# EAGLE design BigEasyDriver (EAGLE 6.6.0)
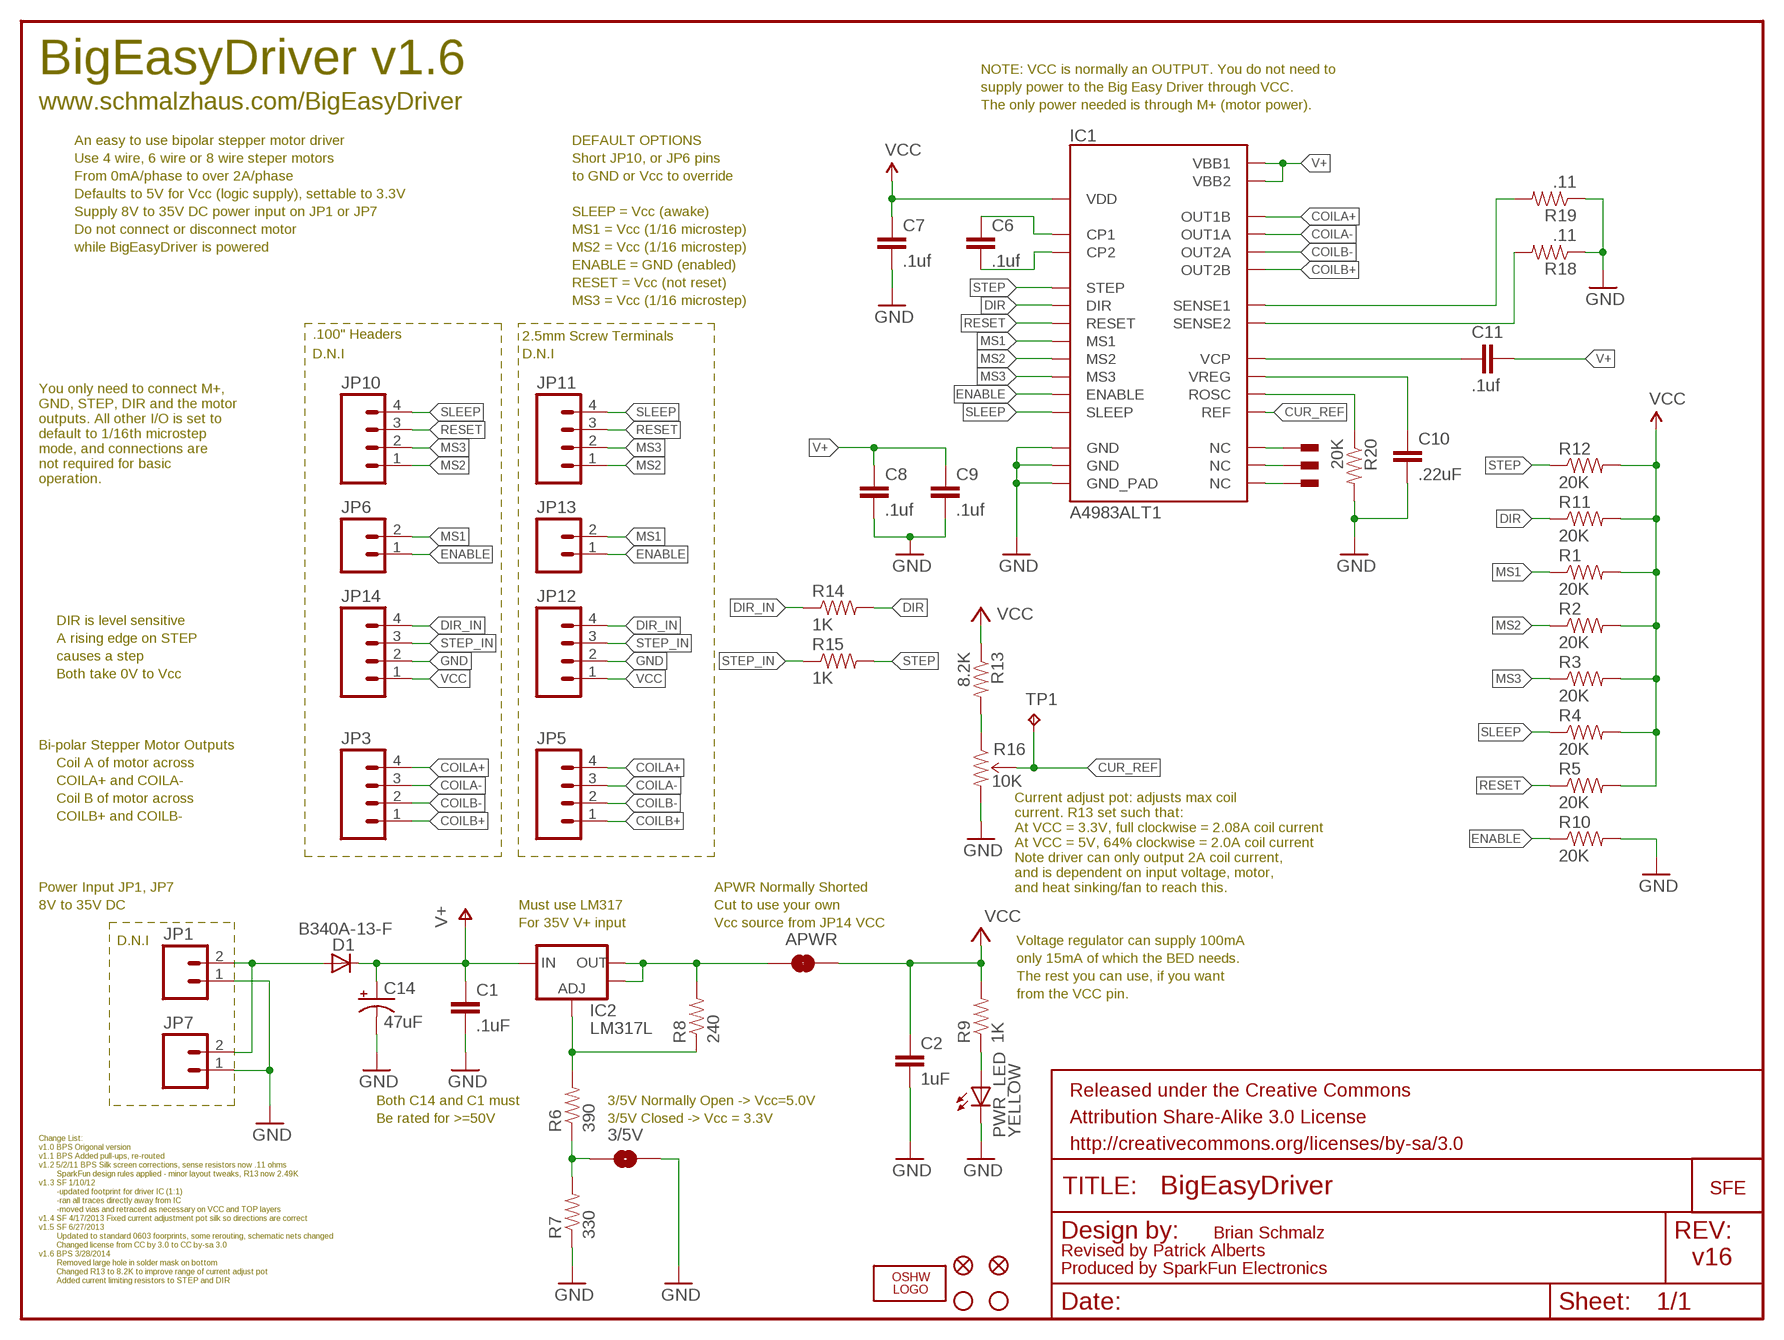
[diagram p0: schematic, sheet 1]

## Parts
3/5V  SOLDERJUMPERNO  [SJ_2S-NO]
APWR  SOLDERJUMPERTRACE  [SJ_2S-TRACE]
C1  .1uF  0.1UF-100V-10%(0603)  [0603-CAP]
C2  1uF  1.0UF-16V-10%(0603)  [0603-CAP]
C6  .1uf  0.1UF-100V-10%(0603)  [0603-CAP]
C7  .1uf  0.1UF-100V-10%(0603)  [0603-CAP]
C8  .1uf  0.1UF-100V-10%(0603)  [0603-CAP]
C9  .1uf  0.1UF-100V-10%(0603)  [0603-CAP]
C10  .22uF  0.22UF50V-20%,+80%(0603)  [0603-CAP]
C11  .1uf  0.1UF-100V-10%(0603)  [0603-CAP]
C14  47uF  47UF-50V-20%(ELECT)  [PANASONIC_D]
D1  B340A-13-F  DIODE-DO-214AC  [DO-214AC]
FID1  FIDUCIAL1X2  [FIDUCIAL-1X2]
FID2  FIDUCIAL1X2  [FIDUCIAL-1X2]
FRAME1  FRAME-LETTER  [CREATIVE_COMMONS]
IC1  A4983ALT1  [QFN-28-5MM_ALT1]
IC2  LM317L  SPARKFUN03_30_09_V_REG_317SOT89SOT89  [SCHMALZHAUS_SOT89]
JP1  M02PTH  [1X02]
JP3  M04PTH  [1X04]
JP5  M04SCREW_LOCK  [SCREWTERMINAL-3.5MM-4_LOCK]
JP6  M02PTH  [1X02]
JP7  M023.5MM_LOCK  [SCREWTERMINAL-3.5MM-2_LOCK]
JP8  STAND-OFF  [STAND-OFF]
JP9  STAND-OFF  [STAND-OFF]
JP10  M04PTH  [1X04]
JP11  M04SCREW_LOCK  [SCREWTERMINAL-3.5MM-4_LOCK]
JP12  M04SCREW_LOCK  [SCREWTERMINAL-3.5MM-4_LOCK]
JP13  M023.5MM_LOCK  [SCREWTERMINAL-3.5MM-2_LOCK]
JP14  M04PTH  [1X04]
LOGO1  OSHW_LOGO_FILLX0100-NT  [OSHW_FILLX100_NOTEXT]
PWR_LED  YELLOW  LED0603  [LED-0603]
R1  20K  20KOHM1/10W5%(0603)  [0603-RES]
R2  20K  20KOHM1/10W5%(0603)  [0603-RES]
R3  20K  20KOHM1/10W5%(0603)  [0603-RES]
R4  20K  20KOHM1/10W5%(0603)  [0603-RES]
R5  20K  20KOHM1/10W5%(0603)  [0603-RES]
R6  390  390OHM1/10W1%(0603)  [0603-RES]
R7  330  330OHM1/10W1%(0603)  [0603-RES]
R8  240  240OHM1/10W1%(0603)  [0603-RES]
R9  1K  1KOHM1/10W1%(0603)  [0603-RES]
R10  20K  20KOHM1/10W5%(0603)  [0603-RES]
R11  20K  20KOHM1/10W5%(0603)  [0603-RES]
R12  20K  20KOHM1/10W5%(0603)  [0603-RES]
R13  8.2K  8.2KOHM-1/10W-5%(0603)  [0603-RES]
R14  1K  1KOHM1/10W1%(0603)  [0603-RES]
R15  1K  1KOHM1/10W1%(0603)  [0603-RES]
R16  10K  TRIMPOT3MM-2  [TRIMPOT-3MM-2]
R18  .11  0.11OHM1/2W1%(2010)  [R2010]
R19  .11  0.11OHM1/2W1%(2010)  [R2010]
R20  20K  20KOHM1/10W5%(0603)  [0603-RES]
TP1  TPPAD1-13  [P1-13]
U$2  LOGO-SFENEW  [SFE-NEW-WEBLOGO]
U$3  PAD  [PAD-0.008]
U$4  PAD  [PAD-0.008]
U$5  PAD  [PAD-0.008]

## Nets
5V_ALT: APWR.1 IC2.OUT IC2.OUT@1(OUT) R8.2
COILA+: IC1.P$21(OUT1B) JP3.4 JP5.4
COILA-: IC1.P$24(OUT1A) JP3.3 JP5.3
COILB+: IC1.P$1(OUT2B) JP3.1 JP5.1
COILB-: IC1.P$26(OUT2A) JP3.2 JP5.2
CUR_REF: IC1.P$17(REF) R16.2(WIPER) TP1.TP
DIR: IC1.P$19(DIR) R11.1 R14.2
DIR_IN: JP12.4 JP14.4 R14.1
ENABLE: IC1.P$2(ENABLE) JP6.1 JP13.1 R10.1
GND: 3/5V.2 C1.2 C2.2 C7.2 C8.2 C9.2 C10.2 C14.- IC1.P$3(GND) IC1.P$18(GND) IC1.P$29(GND_PAD) JP1.1 JP7.1 JP12.2 JP14.2 PWR_LED.C R7.1 R10.2 R16.3(CW) R18.1 R19.1 R20.2
MS1: IC1.P$9(MS1) JP6.2 JP13.2 R1.1
MS2: IC1.P$10(MS2) JP10.1 JP11.1 R2.1
MS3: IC1.P$11(MS3) JP10.2 JP11.2 R3.1
N$1: D1.A JP1.2 JP7.2
N$2: PWR_LED.A R9.1
N$3: R13.2 R16.1(CCW)
N$4: 3/5V.1 R6.1 R7.2
N$5: IC1.P$7(NC) U$3.P$1
N$6: IC2.ADJ R6.2 R8.1
N$7: IC1.P$20(NC) U$4.P$1
N$8: C6.1 IC1.P$4(CP1)
N$9: C6.2 IC1.P$5(CP2)
N$10: IC1.P$25(NC) U$5.P$1
N$19: IC1.P$13(ROSC) R20.1
N$20: C10.1 IC1.P$8(VREG)
N$21: C11.1 IC1.P$6(VCP)
N$31: IC1.P$27(SENSE2) R18.2
N$32: IC1.P$23(SENSE1) R19.2
RESET: IC1.P$12(RESET) JP10.3 JP11.3 R5.1
SLEEP: IC1.P$14(SLEEP) JP10.4 JP11.4 R4.1
STEP: IC1.P$16(STEP) R12.1 R15.2
STEP_IN: JP12.3 JP14.3 R15.1
V+: C1.1 C8.1 C9.1 C11.2 C14.+ D1.C IC1.P$22(VBB1) IC1.P$28(VBB2) IC2.IN
VCC: APWR.2 C2.1 C7.1 IC1.P$15(VDD) JP12.1 JP14.1 R1.2 R2.2 R3.2 R4.2 R5.2 R9.2 R11.2 R12.2 R13.1

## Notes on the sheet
- BigEasyDriver v1.6 | NOTE: VCC is normally an OUTPUT. You do not need to
- supply power to the Big Easy Driver through VCC.
- www.schmalzhaus.com/BigEasyDriver | The only power needed is through M+ (motor power).
- An easy to use bipolar stepper motor driver | DEFAULT OPTIONS
- Use 4 wire, 6 wire or 8 wire steper motors | Short JP10, or JP6 pins
- From 0mA/phase to over 2A/phase | to GND or Vcc to override
- Defaults to 5V for Vcc (logic supply), settable to 3.3V
- Supply 8V to 35V DC power input on JP1 or JP7 | SLEEP = Vcc (awake)
- Do not connect or disconnect motor | MS1 = Vcc (1/16 microstep)
- while BigEasyDriver is powered | MS2 = Vcc (1/16 microstep)
- ENABLE = GND (enabled)
- RESET = Vcc (not reset)
- MS3 = Vcc (1/16 microstep)
- .100" Headers | 2.5mm Screw Terminals
- D.N.I | D.N.I
- You only need to connect M+, 
  GND, STEP, DIR and the motor 
  outputs. All other I/O is set to 
  default to 1/16th microstep 
  mode, and connections are 
  not required for basic 
  operation.
- DIR is level sensitive
- A rising edge on STEP
- causes a step
- Both take 0V to Vcc
- Bi-polar Stepper Motor Outputs
- Coil A of motor across
- COILA+ and COILA-
- Coil B of motor across
- COILB+ and COILB-
- Power Input JP1, JP7 | APWR Normally Shorted
- Current adjust pot: adjusts max coil
  current. R13 set such that:
  At VCC = 3.3V, full clockwise = 2.08A coil current
  At VCC = 5V, 64% clockwise = 2.0A coil current
  Note driver can only output 2A coil current,
  and is dependent on input voltage, motor,
  and heat sinking/fan to reach this.
- 8V to 35V DC | Must use LM317 | Cut to use your own
- For 35V V+ input | Vcc source from JP14 VCC
- D.N.I | Voltage regulator can supply 100mA
- only 15mA of which the BED needs.
- The rest you can use, if you want
- from the VCC pin.
- Both C14 and C1 must | 3/5V Normally Open -> Vcc=5.0V
- Be rated for >=50V | 3/5V Closed -> Vcc = 3.3V
- Change List:
- v1.0 BPS Origonal version
- v1.1 BPS Added pull-ups, re-routed
- v1.2 5/2/11 BPS Silk screen corrections, sense resistors now .11 ohms
- SparkFun design rules applied - minor layout tweaks, R13 now 2.49K
- v1.3 SF 1/10/12
- -updated footprint for driver IC (1:1)
- -ran all traces directly away from IC
- -moved vias and retraced as necessary on VCC and TOP layers
- v1.4 SF 4/17/2013 Fixed current adjustment pot silk so directions are correct
- v1.5 SF 6/27/2013
- Updated to standard 0603 foorprints, some rerouting, schematic nets changed | Brian Schmalz
- Changed license from CC by 3.0 to CC by-sa 3.0
- v1.6 BPS 3/28/2014 | Revised by Patrick Alberts
- Removed large hole in solder mask on bottom | v16
- Changed R13 to 8.2K to improve range of current adjust pot | Produced by SparkFun Electronics
- Added current limiting resistors to STEP and DIR

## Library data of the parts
3/5V APWR = SparkFun03_30_09:SOLDERJUMPER: Solder Jumper
C1 C6-C9 C11 = SparkFun-Capacitors:0.1UF-100V-10%(0603): CAP-08390; PROD_ID: CAP-08390; VALUE: 0.1uF
C2 = SparkFun-Capacitors:1.0UF-16V-10%(0603): CAP-00868; PROD_ID: CAP-00868; VALUE: 1.0uF
C10 = SparkFun-Capacitors:0.22UF50V-20%,+80%(0603): CAP-09885; PROD_ID: CAP-09885; VALUE: 0.22uF
C14 = SparkFun-Capacitors:47UF-50V-20%(ELECT): CAP-10547; PROD_ID: CAP-10547
D1 = diode:DIODE-: DIODE
FID1 FID2 = SparkFun-Aesthetics:FIDUCIAL: Fiducial Alignment Points
FRAME1 = SparkFun-Aesthetics:FRAME-LETTER: Schematic Frame
IC1 = Testing:A4983: DMOS Microstepping Driver with Translator
IC2 = BigEasyDriver_v11:SPARKFUN03_30_09_V_REG_317: Voltage Regulator Standard LM317 adjustable voltage regulator. AOI (Adjust Output Input). Google LM317 Calculator' for easy to use app to get the two resistor values needed. 240/720 for 5V output. 240/390 for 3.3V output. Spark Fun Electronics SKU : COM-00527'
JP1 JP6 = SparkFun:M02: Header 2
JP3 JP10 JP14 = SparkFun:M04: Header 4 Standard 4-pin 0.1" header. Use with straight break away headers (SKU : PRT-00116), right angle break away headers (PRT-00553), swiss pins (PRT-00743), machine pins (PRT-00117), and female headers (PRT-00115). Molex polarized connector foot print use with SKU : PRT-08231 with associated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
JP5 JP11 JP12 = BigEasyDriver_v11:M04: Header 4 Standard 4-pin 0.1" header. Use with straight break away headers (SKU : PRT-00116), right angle break away headers (PRT-00553), swiss pins (PRT-00743), machine pins (PRT-00117), and female headers (PRT-00115). Molex polarized connector foot print use with SKU : PRT-08231 with associated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
JP7 JP13 = BigEasyDriver_v11:M02: Header 2
JP8 JP9 = SparkFun-7-28-09:STAND-OFF: Stand Off
LOGO1 = OSHW:OSHW_LOGO_FILL
PWR_LED = SparkFun03_30_09:LED: LEDs
R1-R5 R10-R12 R20 = SparkFun-Resistors:20KOHM1/10W5%(0603): RES-09231; PROD_ID: RES-09231
R6 = SparkFun-Resistors:390OHM1/10W1%(0603): RES-07864; PROD_ID: RES-07864
R7 = SparkFun-Resistors:330OHM1/10W1%(0603): RES-00818; PROD_ID: RES-00818
R8 = SparkFun-Resistors:240OHM1/10W1%(0603): RES-07849; PROD_ID: RES-07849
R9 R14 R15 = SparkFun-Resistors:1KOHM1/10W1%(0603): RES-07856; PROD_ID: RES-07856
R13 = SparkFun-Resistors:8.2KOHM-1/10W-5%(0603): RES-10646; PROD_ID: RES-10646
R16 = SparkFun-Electromechanical:TRIMPOT: Various small potentiometers for "set-and-forget" applications
R18 R19 = SparkFun-Resistors:0.11OHM1/2W1%(2010): RES-08354; PROD_ID: RES-08354
TP1 = testpad:TP: Test pad
U$2 = SparkFun:LOGO-SFE: Spark Fun Electronics PCB Logo
U$3-U$5 = Testing:PAD

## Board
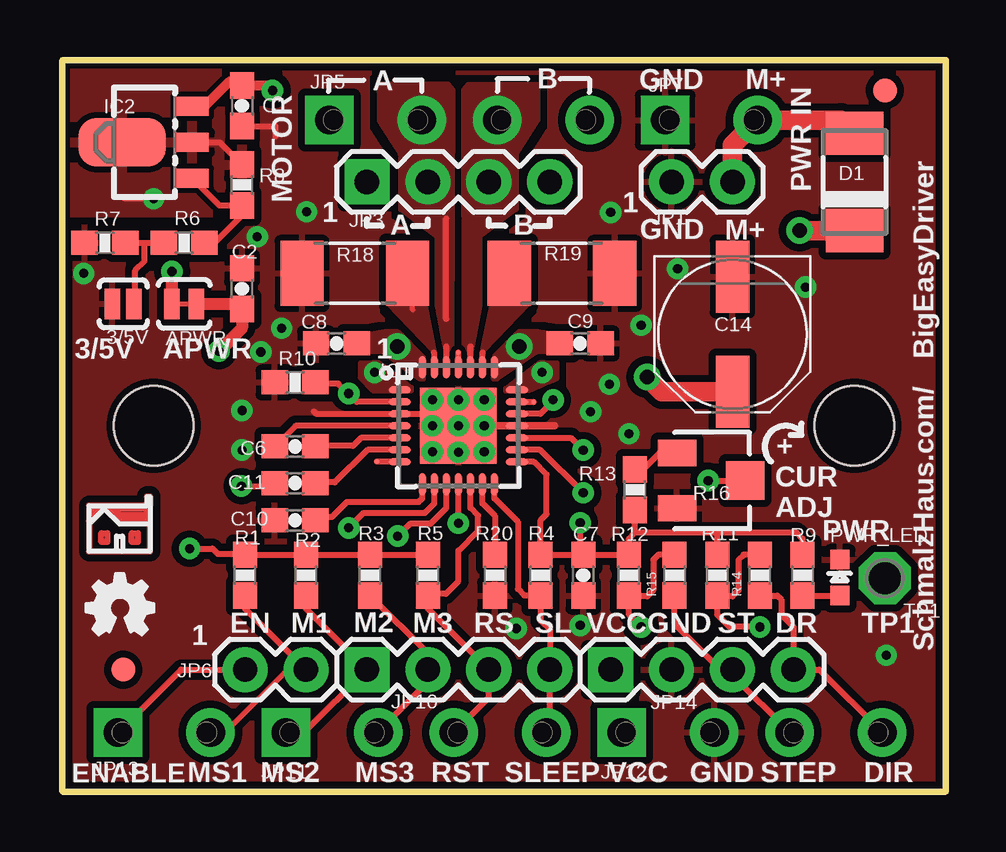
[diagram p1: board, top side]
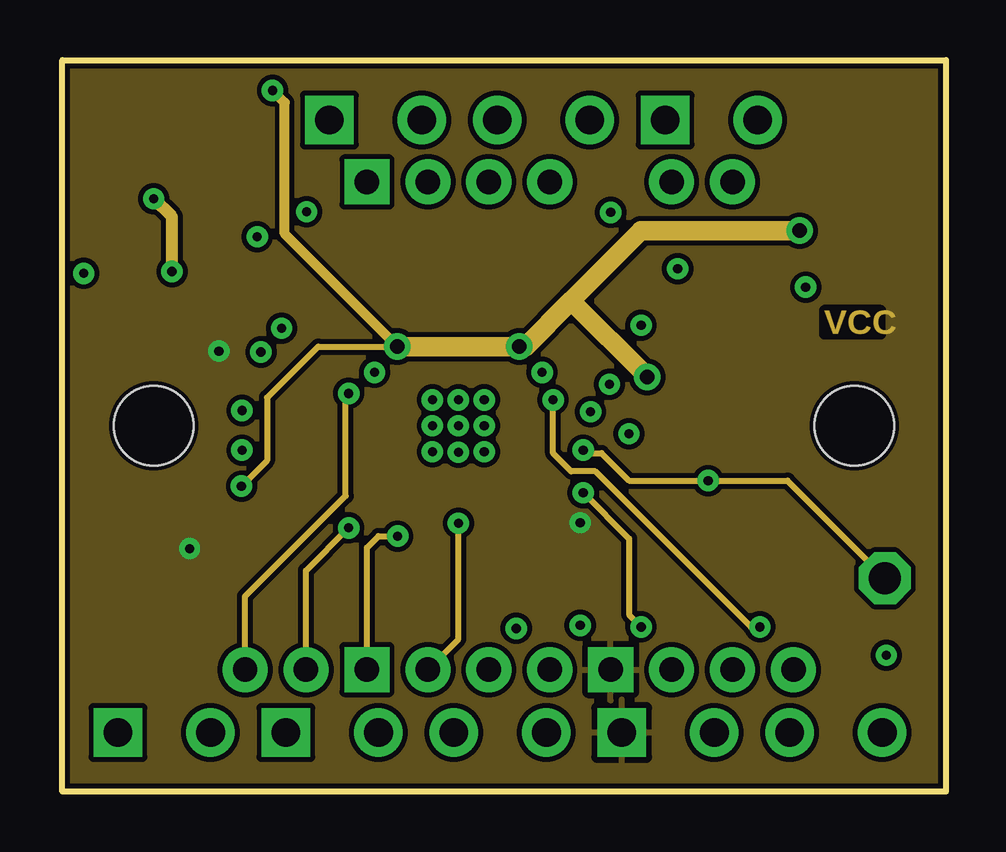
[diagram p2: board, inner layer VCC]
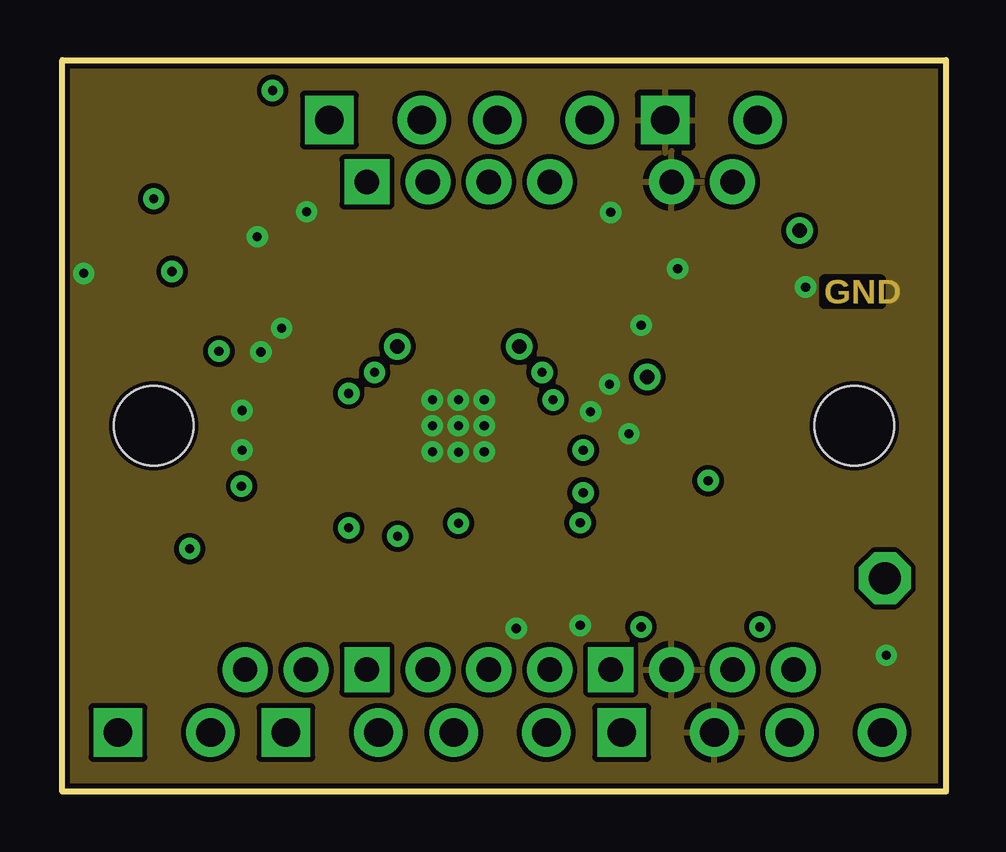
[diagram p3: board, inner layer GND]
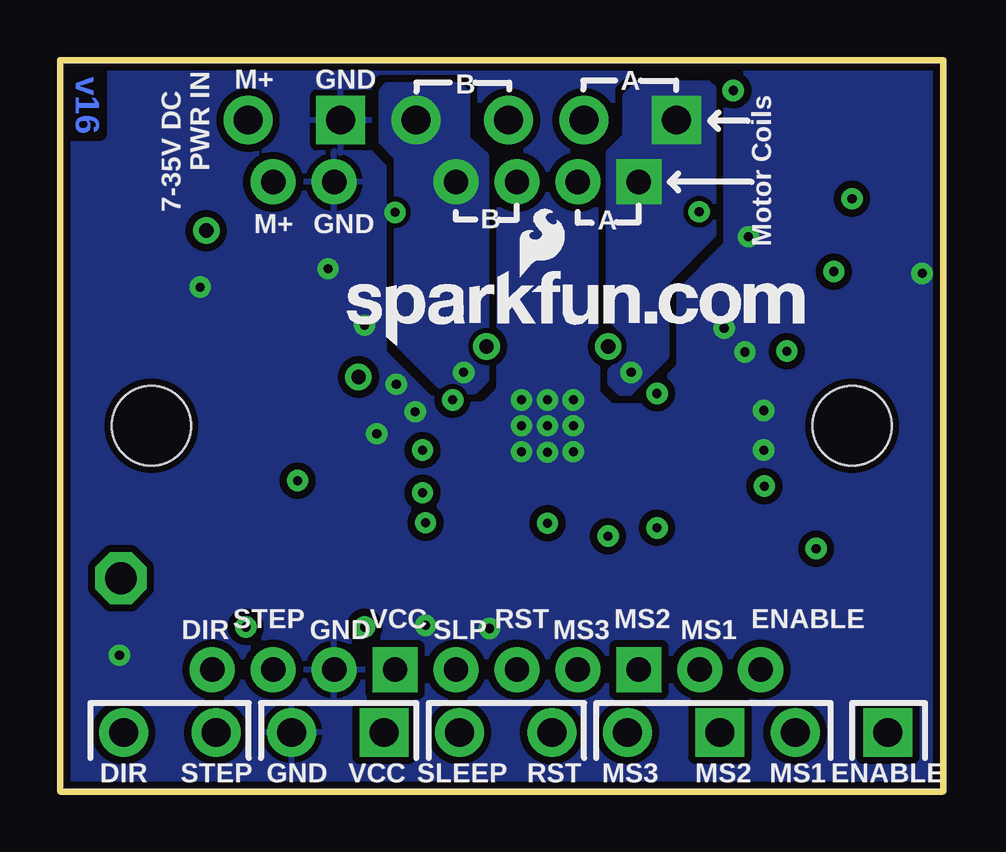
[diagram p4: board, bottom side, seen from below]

Size 36.83 x 30.48 mm. Coordinates in mm from the lower left corner, seen from the top.
Outline: 0,30.48 36.83,30.48 36.83,0 0,0 0,30.48
Copper layers (1*16): Top 0.035mm / dielectric 1.5mm / Bottom 0.035mm
Design rules "SparkFun *": minimum track width 7mil, minimum drill 15mil, track to track 8mil, track to pad 8mil, pad to pad 8mil, via to via 8mil, smd to smd 8mil, copper to edge 8mil, drill to drill 8mil, minimum pad ring 12mil, minimum via ring 10mil, stop-mask expansion 4mil, vias tented up to drill 24mil, thermal gap 10mil

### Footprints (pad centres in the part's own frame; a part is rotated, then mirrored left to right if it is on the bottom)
SJ_2S-NO = smd 0.635 x 1.27: 1 -0.45,0; 2 0.45,0
SJ_2S-TRACE = smd 0.635 x 1.27: 1 -0.508,0; 2 0.508,0
0603-CAP = smd 1.1 x 1: 1 -0.85,0; 2 0.85,0
PANASONIC_D = smd 3 x 1.4: + 2.4,0; - -2.4,0
DO-214AC = smd 1.8 x 2.4: A 2.025,0; C -2.025,0
FIDUCIAL-1X2 = smd 1 x 1: 1 0,0
QFN-28-5MM_ALT1 = smd 0.94 x 0.3: P$1 -2.44,1.5; P$2 -2.44,1; P$3 -2.44,0.5; P$4 -2.44,0; P$5 -2.44,-0.5; P$6 -2.44,-1; P$7 -2.44,-1.5; P$15 2.44,-1.5; P$16 2.44,-1; P$17 2.44,-0.5; P$18 2.44,0; P$19 2.44,0.5; P$20 2.44,1; P$21 2.44,1.5 | smd 0.3 x 0.94: P$8 -1.5,-2.44; P$9 -1,-2.44; P$10 -0.5,-2.44; P$11 0,-2.44; P$12 0.5,-2.44; P$13 1,-2.44; P$14 1.5,-2.44; P$22 1.5,2.44; P$23 1,2.44; P$24 0.5,2.44; P$25 0,2.44; P$26 -0.5,2.44; P$27 -1,2.44; P$28 -1.5,2.44 | smd 3.175 x 3.175: P$29 0,0
SCHMALZHAUS_SOT89 = smd 0.8 x 1.4: ADJ -1.499,-1.981; IN 1.499,-1.981; OUT 0,-1.98 | smd 2.032 x 3.65: OUT@1 0,0.94
1X02 = drill 1.016 pad 1.88: 1 0,0; 2 2.54,0
1X04 = drill 1.016 pad 1.88 square: 1 0,0 | drill 1.016 pad 1.88: 2 2.54,0; 3 5.08,0; 4 7.62,0
SCREWTERMINAL-3.5MM-4_LOCK = drill 1.2 pad 2.032 square: 1 -0.178,0 | drill 1.2 pad 2.032: 2 3.678,0; 3 6.822,0; 4 10.678,0
SCREWTERMINAL-3.5MM-2_LOCK = drill 1.2 pad 2.032 square: 1 -0.178,0 | drill 1.2 pad 2.032: 2 3.678,0
STAND-OFF = hole 3.302: 0,0
LED-0603 = smd 0.8 x 0.8: A 0,-0.75; C 0,0.75
0603-RES = smd 1.1 x 1: 1 -0.85,0; 2 0.85,0
TRIMPOT-3MM-2 = smd 1.092 x 1.6: 1 -1.155,-1.421; 3 1.155,-1.421 | smd 1.6 x 1.6: 2 0,1.421
R2010 = smd 1.8 x 2.7: 1 -2.2,0; 2 2.2,0
P1-13 = drill 1.321 pad 2.159 octagon: TP 0,0
PAD-0.008 = smd 0.203 x 0.203: P$1 0,0

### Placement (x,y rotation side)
3/5V  2.54,20.32 180 top
APWR  5.08,20.32 0 top
C1  7.49,28.57 270 top
C2  7.49,20.95 90 top
C6  9.7,14.38 0 top
C7  21.72,9.02 270 top
C8  11.43,18.67 180 top
C9  21.59,18.67 0 top
C10  9.7,11.3 180 top
C11  9.7,12.85 180 top
C14  27.94,19.05 270 top
D1  33.02,25.4 90 top
FID1  2.54,5.08 0 top
FID2  34.29,29.21 0 top
FRAME1  not placed on the board
IC1  16.51,15.24 0 top
IC2  3.43,27.05 90 top
JP1  25.4,25.4 0 top
JP3  12.7,25.4 0 top
JP5  11.31,27.98 0 top
JP6  7.62,5.08 0 top
JP7  25.31,27.98 0 top
JP8  3.81,15.24 0 top
JP9  33.02,15.24 0 top
JP10  12.7,5.08 0 top
JP11  9.5,2.46 0 top
JP12  23.5,2.46 0 top
JP13  2.5,2.46 0 top
JP14  22.86,5.08 0 top
LOGO1  0.99,6.53 0 top
PWR_LED  32.41,8.92 0 top
R1  7.62,9.02 90 top
R2  10.16,9.02 90 top
R3  12.83,9.02 90 top
R4  19.94,9.02 90 top
R5  15.24,9.02 90 top
R6  5.08,22.86 0 top
R7  1.78,22.86 0 top
R8  7.49,25.27 90 top
R9  30.86,9.02 90 top
R10  9.7,17.04 180 top
R11  27.3,9.02 90 top
R12  23.62,9.02 90 top
R13  23.88,12.57 90 top
R14  29.08,9.02 90 top
R15  25.53,9.02 90 top
R16  27.05,12.95 270 top
R18  12.19,21.59 0 top
R19  20.83,21.59 180 top
R20  18.03,9.02 270 top
TP1  34.29,8.89 0 top
U$1  [SCHMALZHAUS_SMALL]  2.39,10.01 0 top
U$2  24.87,18.57 0 bottom
U$3  13.11,13.74 0 top
U$4  19.66,16.23 0 top
U$5  16.51,18.29 0 top

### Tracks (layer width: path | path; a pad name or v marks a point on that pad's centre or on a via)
5V_ALT  (via drill 0.38)
  Top 0.254: v3.81,24.7 2.6,24.7 2.54,24.77 | IC2.OUT 6.57,27.05 R8.2
  Top 0.508: APWR.1 v4.57,21.67
  VCC 0.508: v4.57,21.67 4.57,23.94 v3.81,24.7
  pour Top: 7.62,30.48 0,30.48 0,24.13 7.62,24.13
COILA+  (via drill 0.38)
  other vias: 20,17.46
  pour Bottom (isolate 0.203, no thermals): 19.05,17.78 19.05,17.14 19.56,16.64 20.76,16.64 22.8,18.67 22.8,26.42 23.43,27.05 23.43,29.21 23.18,29.49 20.13,29.46 19.84,29.1 19.84,27.24 19.05,26.53 19.05,17.84 19.11,17.78
  pour Top (isolate 0.203, no thermals): 18.47,16.79 18.47,16.69 19.46,16.71 20.62,17.22 20.62,17.86 19.89,17.86
COILA-
  Top 0.254: IC1.P$24 17.01,18.53 17.02,18.54
  pour Top (isolate 0.203, no thermals): 16.94,29.48 19.81,29.48 19.81,27.97 18.92,26.54 18.92,24.26 17.4,23.11 17.4,20.24 17.04,18.34 17.04,18.21 16.97,18.21 16.97,18.34 16.76,18.59 16.74,29.24
COILB+  (via drill 0.38)
  other vias: 13.02,17.46
  pour Top (isolate 0.203, no thermals): 12.42,17.86 12.42,17.25 12.94,16.7 14.57,16.7 14.57,16.83 13.21,17.86
  pour Bottom (isolate 0.203, no thermals): 9.59,29.35 9.59,23.18 11.56,21.21 11.56,18.1 13.08,16.57 13.46,16.57 13.91,17.02 13.91,17.53 13.21,18.22 13.21,18.99 13.97,19.75 13.97,26.63 13.27,27.33 13.27,28.99 12.74,29.53 9.8,29.54
COILB-
  Top 0.254: 16,19.68 16,23.88 | IC1.P$26 16.01,18.53 16,18.54
  pour Top (isolate 0.203, no thermals): 16.1,29.46 13.21,29.46 13.21,27.94 14.1,26.54 14.1,24.26 15.62,23.11 15.62,20.27 15.98,18.39 15.98,18.19 16.05,18.19 16.05,18.34 16.26,18.59 16.28,29.24
CUR_REF  (via drill 0.38)
  Top 0.254: v26.92,12.95 R16.2 | IC1.P$17 21.2,14.74 v21.72,14.22
  VCC 0.254: TP1.TP 30.23,12.95 v26.92,12.95 23.62,12.95 22.48,14.1 21.84,14.1 v21.72,14.22
DIR  (via drill 0.38)
  Top 0.254: IC1.P$19 19.93,15.74 20.46,16.27 v20.46,16.32 | R14.2 28.41,9.87 28.19,9.65 28.19,8.38 27.94,8.13 27.34,8.13 R11.1 27.3,7.37 27.81,6.86 v29.08,6.86
  VCC 0.254: v20.46,16.32 20.46,14.08 21.21,13.34 22.23,13.34 28.7,6.86 v29.08,6.86
DIR_IN
  Top 0.254: R14.1 29.81,8.17 29.97,8 29.97,7.37 30.48,6.86 JP14.4 31.56,5.08 JP12.4
ENABLE  (via drill 0.38)
  Top 0.254: JP13.1 2.32,2.45 4.95,5.08 JP6.1 | R10.1 10.6,16.99 11.51,16.99 11.91,16.59 v11.94,16.59 12.28,16.24 IC1.P$2
  VCC 0.254: JP6.1 7.62,8.13 11.81,12.32 11.81,16.46 v11.94,16.59
GND  (via drill 0.38)
  Top 0.254: 15.3,15.75 15.3,15.74 | 8.89,27.3 8.88,27.29 8.88,27.73 C1.2 | 15.3,15.75 15.3,15.37 v15.43,15.24 15.43,15.74 IC1.P$3 | 15.3,15.75 15.3,15.77 | 10.49,15.82 10.57,15.75 14.22,15.75
  Top 0.305: v17.59,15.24 IC1.P$18 20.51,15.24
  other vias: 15.43,16.32 16.51,16.32 17.59,16.32 16.51,15.24 15.43,14.16 16.51,14.14 17.59,14.16 22.81,16.97 30.99,21.02 25.65,21.78 8.13,23.11 0.89,21.59 18.92,6.79 21.59,6.92 34.35,5.68 8.28,18.31 7.49,15.88 24.13,19.43 10.19,24.16 9.14,19.3 7.49,14.22 22.02,15.82 23.62,14.91 22.86,24.13
  pour Top (isolate 0.305, rank 3): 0,30.48 36.83,30.48 36.83,0 0,0
  pour Bottom (isolate 0.305, rank 3): 0,30.48 36.83,30.48 36.83,0 0,0
  pour GND: 0,30.48 36.83,30.48 36.83,0 0,0
MS1  (via drill 0.38)
  Top 0.203: 6.78,2.46 9.4,5.08
  Top 0.254: R1.1 7.62,7.62 JP6.2 9.4,5.08 | JP13.2 6.78,2.46 | IC1.P$9 15.51,12.01 15.11,11.61 12.56,11.61 v11.94,10.99
  VCC 0.254: JP6.2 10.16,9.21 v11.94,10.99
MS2  (via drill 0.38)
  Top 0.254: JP11.1 10.08,2.46 JP10.1 10.16,7.62 R2.1 | IC1.P$10 16.01,11.81 16,11.81 15.34,11.15 14.49,11.15 v13.98,10.64 14.19,10.85
  VCC 0.254: JP10.1 12.7,10.16 13.18,10.64 v13.98,10.64
MS3  (via drill 0.38)
  Top 0.254: JP11.2 13.18,2.51 15.24,4.57 JP10.2 15.24,5.75 R3.1 | v16.51,11.18 IC1.P$11
  VCC 0.254: v16.51,11.18 16.51,6.35 JP10.2
N$1
  Top 0.813: D1.A 32.47,27.98 JP7.2 27.94,26.93 JP1.2
N$2
  Top 0.254: R9.1 PWR_LED.A
N$3
  Top 0.254: R13.2 24.22,13.42 24.89,14.1 25.62,14.1 R16.1
N$4
  Top 0.254: 3/5V.1 3.05,20.32 3.05,21.72 3.43,22.1 3.43,22.86 | R7.2 3.43,22.86 | 3.43,22.86 R6.1
N$5
  Top 0.254: IC1.P$7 U$3.P$1
N$6
  Top 0.254: R6.2 6.35,22.86 7.49,24 R8.1 6.54,24.42 IC2.ADJ
N$7
  Top 0.254: IC1.P$20 U$4.P$1
N$8
  Top 0.254: IC1.P$4 9.72,15.24 C6.1
N$9
  Top 0.254: IC1.P$5 12.45,14.74 12.12,14.4 10.58,14.4 C6.2
N$10
  Top 0.254: IC1.P$25 U$5.P$1
N$19
  Top 0.254: IC1.P$13 17.51,12.01 18.03,11.48 R20.1
N$20
  Top 0.254: IC1.P$8 15.01,12.22 14.86,12.06 11.86,12.06 11.23,11.43 10.68,11.43 C10.1
N$21
  Top 0.254: IC1.P$6 12.72,14.24 11.35,12.88 10.58,12.88 C11.1
N$31
  Top 0.203: 14.61,20.07 14.61,21.3
  Top 0.254: R18.2 13.97,21.59 | IC1.P$27 15.51,18.27 15.49,18.29
  pour Top (isolate 0.203, no thermals): 13.59,20.32 15.48,18.34 15.48,18.17 15.54,18.2 15.11,20.32
N$32
  Top 0.254: IC1.P$23 17.51,18.27 17.53,18.29
  pour Top (isolate 0.203, no thermals): 17.48,18.21 17.55,18.21 17.55,18.36 19.43,20.32 17.91,20.32
RESET
  Top 0.254: JP11.3 16.32,2.48 17.78,3.94 JP10.3 15.24,7.62 R5.1 15.31,8.24 15.99,8.24 16.51,8.76 16.51,10.03 17.34,10.86 17.34,11.49 17.01,11.82 IC1.P$12
SLEEP
  Top 0.254: JP11.4 20.32,2.6 JP10.4 20.32,6.73 19.94,7.11 R4.1 19.27,8.17 18.99,8.45 18.99,11.24 18.01,12.22 IC1.P$14
STEP  (via drill 0.38)
  Top 0.254: IC1.P$16 19.92,14.24 v21.72,12.45 | R15.2 24.85,9.87 24.64,9.65 24.64,8.38 24.38,8.13 23.66,8.13 R12.1 23.62,7.37 v24.13,6.86
  VCC 0.254: v21.72,12.45 23.62,10.54 23.62,7.37 v24.13,6.86
STEP_IN
  Top 0.254: R15.1 25.53,6.99 27.43,5.08 JP14.3 27.94,4.84 JP12.3
V+  (via drill 0.38, 0.6)
  Top 0.203: IC1.P$28 15.01,18.01
  Top 0.254: IC1.P$22 18.01,18.01 | v7.47,12.72 8.73,12.72 C11.2
  Top 0.406: 8.76,29.08 v8.76,29.21 8.55,29.43 C1.1 7.33,29.59 6.99,29.59 5.94,28.55 IC2.IN
  Top 0.813: D1.C v30.74,23.38 v30.73,23.37 | C14.+ 25.01,16.65 v24.38,17.27
  VCC 0.254: v13.97,18.54 10.67,18.54 8.53,16.41 8.53,13.79 v7.47,12.72
  VCC 0.406: v8.76,29.21 9.27,28.7 9.27,23.24 v13.97,18.54
  VCC 0.813: v30.73,23.37 24.13,23.37 21.21,20.45 | 21.21,20.45 19.3,18.54 v19.05,18.54 v13.97,18.54 | 21.21,20.45 v24.38,17.27
  pour Top (isolate 0.203, no thermals): 12.37,18.31 12.37,19 13.46,19.18 13.97,19.18 15.06,18.07 15.06,17.18 14.9,17.18 13.36,18.31
  pour Top (isolate 0.203, no thermals): 18.03,18.16 19.05,19.18 19.81,19.18 20.6,19.05 20.6,18.29 19.79,18.31 18.11,17.17 17.98,17.17
VCC  (via drill 0.38)
  Top 0.254: 23.88,10.79 27.3,10.79 | R5.2 R3.2 R2.2 R1.2 7.58,9.91 6.48,9.91 6.26,10.12 v5.31,10.12 | 21.59,9.87 R4.2 19.94,11.3 20.19,11.56 20.19,13.21 19.66,13.74 IC1.P$15 | 21.59,9.87 C7.1 R12.2 23.62,10.54 23.88,10.79 | R11.2 27.3,10.79 | 27.3,10.79 30.61,10.79 30.86,10.54 R9.2 | v21.59,11.2 21.59,9.87 | 23.88,10.79 R13.1
  Top 0.508: APWR.2 7.28,20.32 C2.1 7.49,19.32 v6.53,18.35
  pour VCC: 0,30.48 36.83,30.48 36.83,0 0,0

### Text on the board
VCC: VCC
GND: GND
Bottom: v16
tPlace: A | B | GND | M+ | MOTOR | PWR IN | 1 | 1 | A | B | GND | M+ | 3/5V | APWR | 1 | BigEasyDriver | + | CUR | ADJ | PWR | EN | M1 | M2 | M3 | RS | SL | VCC | GND | ST | DR | TP1 | 1 | SchmalzHaus.com/ | ENABLE | MS1 | MS2 | MS3 | RST | SLEEP | VCC | GND | STEP | DIR
bPlace: A | B | GND | M+ | PWR IN | 7-35V DC | Motor Coils | A | B | GND | M+ | ENABLE | MS2 | RST | VCC | STEP | MS1 | MS3 | SLP | GND | DIR | ENABLE | MS1 | MS2 | MS3 | RST | SLEEP | VCC | GND | STEP | DIR
tValues: Brian Schmalz: http://schmalzhaus.com/BigEasyDriver/index.html
tDocu: THIS IS A 4-LAYER BOARD. | Revised by: Patrick Alberts/Toni Klopfenstein | Produced by SparkFun Electronics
